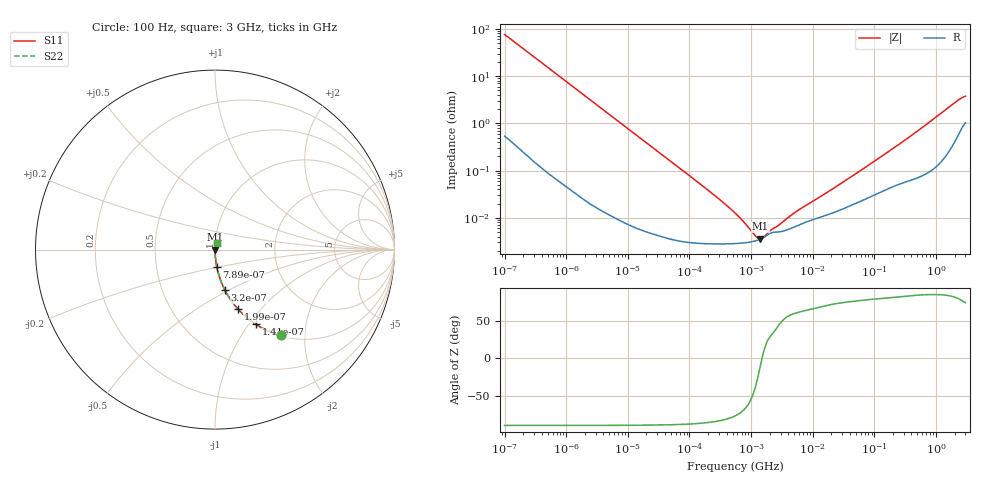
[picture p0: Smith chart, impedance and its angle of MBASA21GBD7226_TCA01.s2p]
! MBASA21GBD7226_TCA01  S-PARAMETER MODEL  ( Standard Model )
! Model Generated by TAIYO YUDEN Corporation (http://www.ty-top.com)
! Version 1.0
! TAIYO YUDEN Control No. 231201
! Copyright(c) 2023 TAIYO YUDEN CO.,LTD. All Rights Reserved.
! Product Description (link to TY-COMPAS)
! https://ds.yuden.co.jp/TYCOMPAS/or/detail?pn=MBASA21GBD7226MTCA01&u=M
! Products Name : Multilayer Ceramic Capacitors
! Characteristics :
!  Capacitance : 22 [uF] , Rated Voltage : 4 [V] , TCC : X7T
!  Case Size : 2.0 x 1.25 / 0.079 x 0.049 [mm/inch] , Thickness : 1.25 / 0.049 [mm/inch]
!  (Conditions: Temperature = 25 [degC] , DC Bias Voltage = 0 [V])
! External Node Assignments :
!  1  o---| |---o  2
! GND o---------o GND
! Frequency Range : 100Hz  -  3GHz  [ 401 STEP ]
# MHZ S RI R 50
! Freq[MHz].  S11 Real  S11 Imag  S21 Real  S21 Imag  S12 Real  S12 Imag  S22 Real  S22 Imag
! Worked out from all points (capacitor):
!   401 points, 100 Hz to 3 GHz, reference 50 ohm
!   read as one part in series: C = 20.9 uF near 109 Hz
!   lowest |Z| = 3.59 mohm at 1.412 MHz (marker M1)
!   series resonance near 1.505 MHz, so ESL is about 540 pH
!   S11 on the Smith chart (normalised r, x): 100 Hz: 1.01, -1.52; 141 Hz: 1.01, -1.08; 199 Hz: 1.00, -0.77; 320 Hz: 1.00, -0.48; 789 Hz: 1.00, -0.19; 3 GHz: 1.02, +0.07
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0.0001  0.3672 -0.4785  0.6328 0.4785  0.6328 0.4785  0.3672 -0.4785
0.000141  0.2272 -0.4156  0.7728 0.4156  0.7728 0.4156  0.2272 -0.4156
0.000199  0.1296 -0.3327  0.8704 0.3327  0.8704 0.3327  0.1296 -0.3327
0.00032  0.0553 -0.2255  0.9447 0.2255  0.9447 0.2255  0.0553 -0.2255
0.000513  0.0226 -0.1456  0.9774 0.1456  0.9774 0.1456  0.0226 -0.1456
0.000789  0.00989 -0.0961  0.9901 0.0961  0.9901 0.0961  0.00989 -0.0961
0.001788  0.0021 -0.0429  0.9979 0.0429  0.9979 0.0429  0.0021 -0.0429
0.005476  0.000306 -0.0141  0.9997 0.0141  0.9997 0.0141  0.000306 -0.0141
0.031977  4.72e-05 -0.00243  1 0.00243  1 0.00243  4.72e-05 -0.00243
0.231582  2.82e-05 -0.000329  1 0.000329  1 0.000329  2.82e-05 -0.000329
0.547723  2.85e-05 -0.000124  1 0.000124  1 0.000124  2.85e-05 -0.000124
0.623217  2.87e-05 -0.000104  1 0.000104  1 0.000104  2.87e-05 -0.000104
0.709116  2.91e-05 -8.55e-05  1 8.55e-05  1 8.55e-05  2.91e-05 -8.55e-05
1.411895  3.54e-05 -6.37e-06  1 6.37e-06  1 6.37e-06  3.54e-05 -6.37e-06
3.79959  5.52e-05 7.89e-05  0.9999 -7.89e-05  0.9999 -7.89e-05  5.52e-05 7.89e-05
9.794414  9.03e-05 0.000201  0.9999 -0.000201  0.9999 -0.000201  9.03e-05 0.000201
32.68714  0.000159 0.000574  0.9998 -0.000574  0.9998 -0.000574  0.000159 0.000574
175.1444  0.000429 0.00256  0.9996 -0.00256  0.9996 -0.00256  0.000429 0.00256
492.0662  0.000739 0.0067  0.9993 -0.0067  0.9993 -0.0067  0.000739 0.0067
2126.076  0.00541 0.0283  0.9946 -0.0283  0.9946 -0.0283  0.00541 0.0283
2636.591  0.00899 0.0333  0.991 -0.0333  0.991 -0.0333  0.00899 0.0333
3000  0.0114 0.0353  0.9886 -0.0353  0.9886 -0.0353  0.0114 0.0353
